TYPE ST_event :
STRUCT
	severity : INT := 0; // 0 - info, 1 - warning, 2 - error, 3 - critical
	state : INT := 0; // 0 - inactive, 1 - raised, 2 - confirmed, 3 - active (non-confirmable)
	needs_confirmation : BOOL := FALSE; // FALSE: INACTIVE -> ACTIVE; we go to INACTIVE after received clear action; TRUE: when in state RAISED, we go to CONFIRMED after confirm action, and then to INACTIVE after clear
	timestamp_raised : DATE_AND_TIME; // When event was raised
	timestamp_confirmed : DATE_AND_TIME; // When event was confirmed
	display_text : STRING(255) := '';
	cause_text : STRING(255) := '';
	remedy_text : STRING(255) := '';	
END_STRUCT
END_TYPE
